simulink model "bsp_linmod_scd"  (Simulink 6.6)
settings: Solver=ode45  StartTime=0.0  StopTime=0.5  RelTol=1e-3

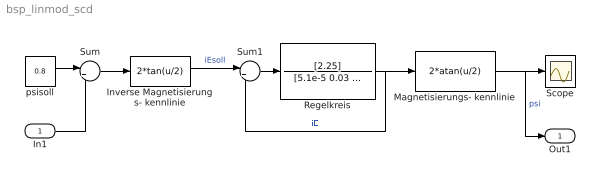
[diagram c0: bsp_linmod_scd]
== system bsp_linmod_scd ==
  In1 : Inport
  Inverse Magnetisierungs- kennlinie : Fcn  Expr=2*tan(u/2)
  Magnetisierungs- kennlinie : Fcn  Expr=2*atan(u/2)
  Regelkreis : TransferFcn  Numerator=[2.25]  Denominator=[5.1e-5 0.03 0]
  Scope : Scope
  Sum : Sum  Inputs=|++
  Sum1 : Sum  Inputs=|+-
  psisoll : Constant  Value=0.8
  Out1 : Outport
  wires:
  Inverse Magnetisierungs- kennlinie/1 -> Sum1/1  "iEsoll"
  Sum1/1 -> Regelkreis/1
  Magnetisierungs- kennlinie/1 -> Scope/1, Out1/1  "psi"
  Regelkreis/1 -> Magnetisierungs- kennlinie/1, Sum1/2  "iE"
  psisoll/1 -> Sum/1
  Sum/1 -> Inverse Magnetisierungs- kennlinie/1
  In1/1 -> Sum/2
